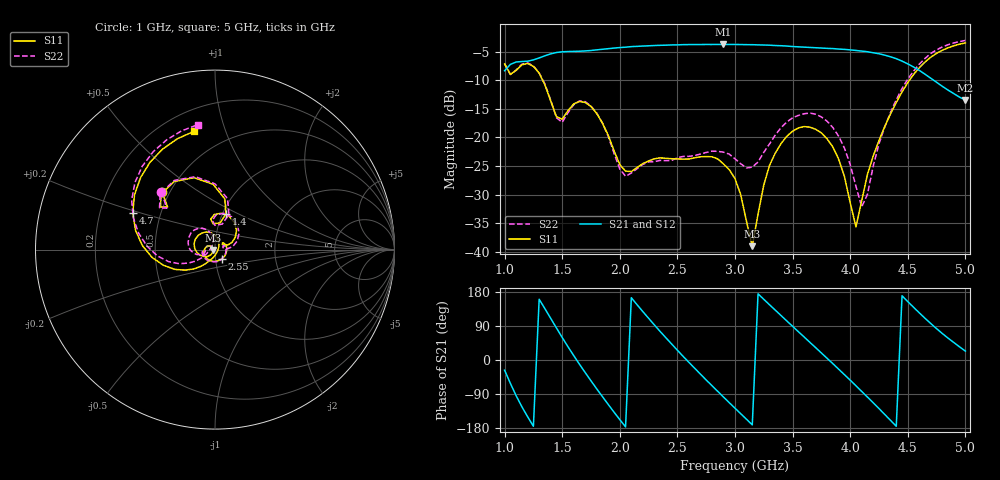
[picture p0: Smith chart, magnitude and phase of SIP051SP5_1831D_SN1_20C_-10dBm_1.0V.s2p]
# GHz  S  dB  R  50
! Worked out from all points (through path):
!   81 points, 1 GHz to 5 GHz, reference 50 ohm
!   highest |S21| = -3.76 dB at 2.9 GHz (marker M1); lowest = -13.5 dB at 5 GHz (marker M2)
!   lowest |S11| = -39.0 dB at 3.15 GHz (marker M3), VSWR 1.02, Z = 48.9 - j0.205 ohm
!   |S11| at or under -10 dB: 1.33 GHz to 4.515 GHz (3.186 GHz wide, 109 % of centre)
!   |S22| runs from -32.2 to -3.1 dB; largest |S21 - S12| = 0.003
!   S11 on the Smith chart (normalised r, x): 1 GHz: 0.45, +0.36; 1.4 GHz: 1.04, +0.43; 2.55 GHz: 1.07, -0.11; 4.7 GHz: 0.34, +0.19; 5 GHz: 0.33, +0.78
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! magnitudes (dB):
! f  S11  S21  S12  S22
! 1 GHz  -7.2  -8.4  -8.3  -7.2
! 1.25 GHz  -7.6  -6.5  -6.5  -7.5
! 1.4 GHz  -13.6  -5.4  -5.4  -13.5
! 1.5 GHz  -16.8  -5.0  -5.0  -17.4
! 1.7 GHz  -13.9  -4.9  -4.9  -13.8
! 1.85 GHz  -17.5  -4.6  -4.6  -17.5
! 2.05 GHz  -25.9  -4.2  -4.2  -26.8
! 2.35 GHz  -23.6  -3.9  -3.9  -24.0
! 2.55 GHz  -23.8  -3.8  -3.8  -23.3
! 2.9 GHz  -24.7  -3.8  -3.8  -22.6
! 3 GHz  -27.2  -3.8  -3.8  -23.8
! 3.15 GHz  -39.0  -3.8  -3.8  -25.2
! 3.25 GHz  -28.3  -3.9  -3.9  -22.6
! 3.35 GHz  -22.8  -4.0  -3.9  -19.6
! 3.5 GHz  -18.9  -4.1  -4.1  -16.6
! 3.7 GHz  -18.6  -4.3  -4.3  -16.0
! 3.9 GHz  -23.8  -4.6  -4.6  -19.8
! 4.05 GHz  -35.7  -4.8  -4.8  -28.6
! 4.1 GHz  -31.1  -4.9  -4.9  -32.2
! 4.35 GHz  -15.9  -5.9  -5.9  -15.7
! 4.7 GHz  -6.0  -9.7  -9.7  -5.3
! 5 GHz  -3.5  -13.5  -13.4  -3.1
